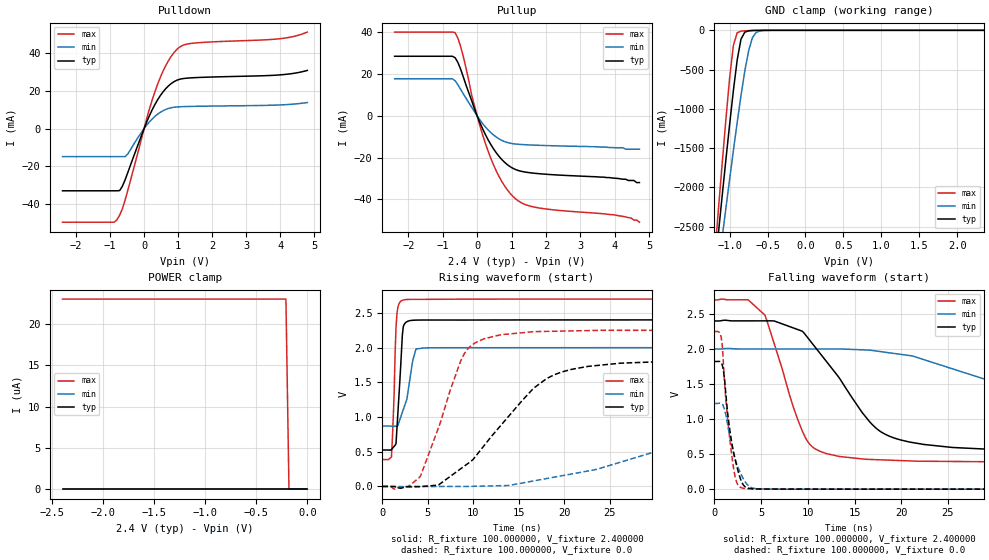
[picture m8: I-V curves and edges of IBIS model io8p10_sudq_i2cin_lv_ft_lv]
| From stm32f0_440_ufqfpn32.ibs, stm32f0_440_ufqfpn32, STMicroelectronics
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|   Model io8p10_sudq_i2cin_lv_ft_lv
[Model]  io8p10_sudq_i2cin_lv_ft_lv
Model_type I/O
Polarity   Non-Inverting
Enable   Active-Low
Vinl =   0.720000V
Vinh =   1.680000V
Vmeas =  1.200000V
Cref =   50.000000pF
Rref =   100.000000M
Vref =   0.0V
C_comp   2.067900pF   1.988600pF   2.164800pF
[Temperature Range]   25.000000   0.125000k   -40.000000
[Pullup Reference]   2.400000V   2.000000V   2.700000V
[Pulldown Reference]   0.0V   0.0V   0.0V
[POWER Clamp Reference]   2.400000V   2.000000V   2.700000V
[GND Clamp Reference]   0.0V   0.0V   0.0V
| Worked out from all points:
|   slope of the pulldown table from 0 to 0.36 V, typ, clamps not added: 25.5 ohm
|   slope of the pullup table from 0 to 0.36 V, typ, clamps not added: 28.4 ohm
|   GND clamp passes 1 mA (typ) near -0.64 V on its own axis
|   rising waveform, R_fixture 100.000000, V_fixture 2.400000: 20-80 % time 502ps typ, 1.02ns min, 335ps max; typ from 0.525 V to 2.4 V
|   rising waveform, R_fixture 100.000000, V_fixture 0.0: 20-80 % time 7.3ns typ, 20.9ns min, 3.55ns max; typ from 0 V to 1.82 V
|   falling waveform, R_fixture 100.000000, V_fixture 2.400000: 20-80 % time 6.28ns typ, 18ns min, 3.34ns max; typ from 2.4 V to 0.525 V
|   falling waveform, R_fixture 100.000000, V_fixture 0.0: 20-80 % time 1.17ns typ, 1.4ns min, 928ps max; typ from 1.82 V to 0 V
[Pulldown]
|Voltage   I(typ)   I(min)   I(max)
-2.4V     -33.16mA   -14.98mA   -49.86mA
-880mV    -33.16mA   -14.98mA   -49.86mA
-800mV    -33.16mA   -14.98mA   -48.55mA
-640mV    -30.75mA   -14.98mA   -42.76mA
-480mV    -23.43mA   -13.57mA   -32.92mA
80mV      3.651mA    1.905mA    5.506mA
400mV     15.37mA    7.665mA    23.73mA
720mV     22.75mA    10.69mA    36.23mA
1.04V     26.18mA    11.57mA    43.27mA
1.52V     27.09mA    11.81mA    45.55mA
4V        28.55mA    12.55mA    47.81mA
4.8V      30.9mA     13.81mA    51.31mA
[Pullup]
|Voltage   I(typ)   I(min)   I(max)
-2.4V     28.55mA    17.74mA    40.14mA
-720mV    28.55mA    17.74mA    40.14mA
-640mV    27.85mA    16.83mA    39.87mA
-480mV    22.39mA    12.65mA    33.23mA
-80mV     3.427mA    2.067mA    4.957mA
160mV     -6.219mA   -3.714mA   -9.136mA
320mV     -11.51mA   -6.781mA   -16.98mA
720mV     -21mA      -11.8mA    -31.53mA
1.12V     -25.77mA   -13.54mA   -39.82mA
1.76V     -27.69mA   -14.12mA   -44.06mA
4V        -29.9mA    -15.3mA    -47.5mA
4.72V     -32mA      -16mA      -51mA
[GND_clamp]
|Voltage   I(typ)   I(min)   I(max)
-2.4V     -9.567A    -9.921A    -9.731A
-1.2V     -3.09A     -3.428A    -2.911A
-1.15V    -2.606A    -3.04A     -2.31A
-1.1V     -2.127A    -2.655A    -1.719A
-1.05V    -1.657A    -2.274A    -1.146A
-950mV    -765.3mA   -1.53A     -190.2mA
-900mV    -376.6mA   -1.172A    -30.81mA
-850mV    -112.3mA   -832.5mA   -10.23mA
-750mV    -6.57mA    -264.6mA   -4.026mA
-700mV    -2.581mA   -94.26mA   -2.329mA
-600mV    -416.4uA   -8.158mA   -368uA
2.35V     0A         0A         0A
[POWER_clamp]
|Voltage   I(typ)   I(min)   I(max)
-2.4V     0A         0A         23.03uA
-210mV    0A         0A         23.03uA
-180mV    0A         0A         0A
0V        0A         0A         0A
[Ramp]
| variable   typ   min   max
dV/dt_r  1.09308/7.29892n   0.73302/20.91059n   1.34964/3.54172n
dV/dt_f  1.12475/6.26977n   0.67617/18.01379n   1.38754/3.33048n
R_load = 100.000000
[Rising Waveform]
R_fixture= 100.000000
V_fixture= 2.400000
V_fixture_min= 2.000000
V_fixture_max= 2.700000
|time   V(typ)   V(min)   V(max)
0s        525.2mV    870.3mV    387.4mV
1.001ns   533.1mV    868.7mV    426.5mV
1.301ns   578.4mV    867.2mV    1.363V
1.401ns   593.6mV    866.8mV    1.917V
1.502ns   616mV      866.5mV    2.287V
1.702ns   1.045V     876.9mV    2.575V
2.202ns   2.185V     1.069V     2.683V
2.503ns   2.353V     1.185V     2.692V
3.704ns   2.397V     1.982V     2.696V
49.85ns   2.4V       2V         2.7V
[Rising Waveform]
R_fixture= 100.000000
V_fixture= 0.0
V_fixture_min= 0.0
V_fixture_max= 0.0
|time   V(typ)   V(min)   V(max)
0s        1.475nV    15.65nV    1.121nV
2.803ns   -3.421mV   -6.233mV   -1.618mV
4.204ns   -1.817mV   -2.142mV   151.4mV
8.809ns   273mV      -646.9uV   1.865V
10.21ns   426.3mV    2.665mV    2.069V
13.01ns   876.3mV    10.91mV    2.185V
18.22ns   1.564V     117.4mV    2.235V
26.03ns   1.774V     343.1mV    2.249V
51.25ns   1.823V     1.1V       2.249V
99.7ns    1.822V     1.223V     2.249V
[Falling Waveform]
R_fixture= 100.000000
V_fixture= 2.400000
V_fixture_min= 2.000000
V_fixture_max= 2.700000
|time   V(typ)   V(min)   V(max)
0s        2.4V       2V         2.7V
3.604ns   2.401V     2V         2.702V
5.405ns   2.402V     2V         2.483V
9.81ns    2.191V     2V         717.7mV
13.41ns   1.578V     2V         465.8mV
17.82ns   818.7mV    1.962V     418.4mV
25.43ns   595.6mV    1.72V      395.4mV
41.64ns   535.1mV    1.108V     387.6mV
48.85ns   529.2mV    974.3mV    387.3mV
99.7ns    525.2mV    870.3mV    387.4mV
[Falling Waveform]
R_fixture= 100.000000
V_fixture= 0.0
V_fixture_min= 0.0
V_fixture_max= 0.0
|time   V(typ)   V(min)   V(max)
0s        1.822V     1.223V     2.249V
700.7ps   1.802V     1.222V     2.181V
1.001ns   1.657V     1.166V     1.713V
1.401ns   1.1V       927.1mV    1.015V
1.902ns   626.6mV    598.3mV    437.2mV
2.302ns   378mV      394.2mV    128.4mV
2.903ns   106.9mV    196.9mV    19.59mV
3.704ns   11.99mV    41.57mV    4.599mV
4.905ns   2.494mV    3.765mV    2.382mV
49.85ns   1.475nV    15.65nV    1.121nV
